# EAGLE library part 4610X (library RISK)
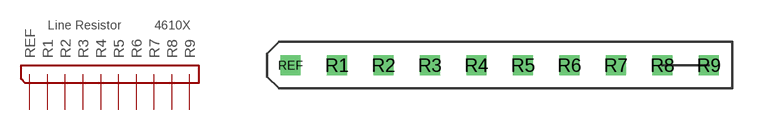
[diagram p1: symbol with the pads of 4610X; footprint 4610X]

Designator prefix -

## 4610X  [4610X]
R1  R1
R2  R2
R3  R3
R4  R4
R5  R5
R6  R6
R7  R7
R8  R8
R9  R9
REF  REF

## Footprint 4610X (pad centres in mm)
drill 0.6 square: R1 -8.89,0; R2 -6.35,0; R3 -3.81,0; R4 -1.27,0; R5 1.27,0; R6 3.81,0; R7 6.35,0; R8 8.89,0; R9 11.43,0; REF -11.43,0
